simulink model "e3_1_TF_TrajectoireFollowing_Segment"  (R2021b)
settings: Solver=FixedStepAuto  StartTime=0.0  StopTime=100  FixedStep=sampleTime  RelTol=1e-3  EnableMultiTasking=on
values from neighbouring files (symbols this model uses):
  k_d_x = 1.5    [startSimulation.m]    (also in StartSimulation.m; start.m = 1.65)
  k_d_y = 1.5    [startSimulation.m]    (also in StartSimulation.m; start.m = 1.52)
  k_d_yaw = 1    [startSimulation.m]    (also in StartSimulation.m; start.m)
  k_d_z = 0.5    [startSimulation.m]    (also in StartSimulation.m; start.m)
  k_i_x = 0.01    [startSimulation.m]    (also in StartSimulation.m; start.m = 0.9)
  k_i_y = 0.01    [startSimulation.m]    (also in StartSimulation.m; start.m = 0.91)
  k_i_yaw = 0.01    [startSimulation.m]    (also in StartSimulation.m; start.m)
  k_i_z = 0.01    [startSimulation.m]    (also in StartSimulation.m; start.m)
  k_p_x = 1.2    [startSimulation.m]    (also in StartSimulation.m; start.m = 1.9)
  k_p_y = 1.5    [startSimulation.m]    (also in StartSimulation.m; start.m = 1.9)
  k_p_yaw = 2    [startSimulation.m]    (also in StartSimulation.m; start.m)
  k_p_z = 2    [startSimulation.m]    (also in StartSimulation.m; start.m)
  saturation_psi = 2    [startSimulation.m]    (also in StartSimulation.m; start.m)
  saturation_x = 2    [startSimulation.m]    (also in StartSimulation.m; start.m)
  saturation_y = 2    [startSimulation.m]    (also in StartSimulation.m; start.m)
  saturation_z = 2    [startSimulation.m]    (also in StartSimulation.m; start.m)
libraries: simulink x28, aerolibanimutils x1

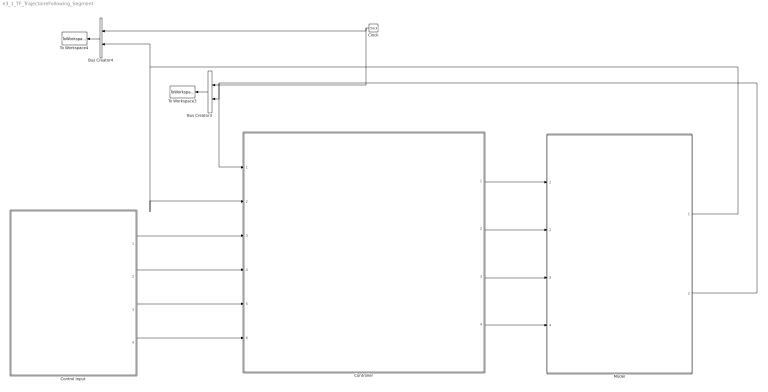
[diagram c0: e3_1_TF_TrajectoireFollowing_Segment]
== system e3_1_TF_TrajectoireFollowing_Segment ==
  Bus Creator3 : BusCreator  Inputs=2
  Bus Creator4 : BusCreator  Inputs=2
  Clock : Clock
  Control Input : Subsystem
  Controller : Subsystem
  Model : Subsystem
  To Workspace3 : ToWorkspace  VariableName=r1_pos_array  SampleTime=-1
  To Workspace4 : ToWorkspace  VariableName=r1_vel_array  SampleTime=-1
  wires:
  Clock/1 -> Bus Creator4/1, Bus Creator3/1
  Bus Creator3/1 -> To Workspace3/1
  Bus Creator4/1 -> To Workspace4/1
  Controller/1(Controller Output X) -> Model/1(Commande Input X)
  Controller/2(Controller Output Y) -> Model/2(Commande Input Y)
  Controller/3(Controller Output H) -> Model/3(Commande Input H)
  Controller/4(Controller Output Psi) -> Model/4(Commande Input Psi)
  Control Input/1(ux) -> Controller/3(Control input X)
  Control Input/2(uy) -> Controller/4(Control input Y)
  Control Input/3(uz) -> Controller/5(Control input H)
  Control Input/4(upsi) -> Controller/6(Control input Psi)
  Model/2(Output Position) -> Controller/1(Feedback Position), Bus Creator3/2
  Model/1(Output Velocity) -> Controller/2(Feedback Velocity), Bus Creator4/2

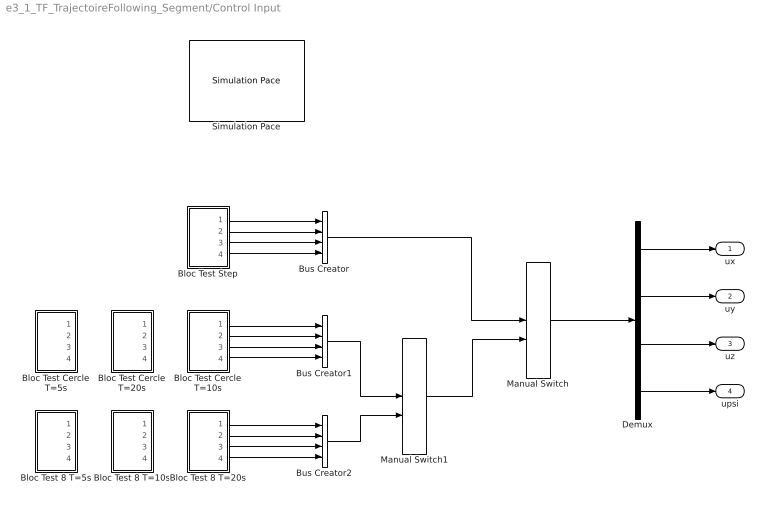
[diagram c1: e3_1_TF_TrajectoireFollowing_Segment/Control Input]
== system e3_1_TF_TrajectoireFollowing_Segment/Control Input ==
  Bloc Test 8 T=10s : Subsystem
  Bloc Test 8 T=20s : Subsystem
  Bloc Test 8 T=5s : Subsystem
  Bloc Test Cercle T=10s : Subsystem
  Bloc Test Cercle T=20s : Subsystem
  Bloc Test Cercle T=5s : Subsystem
  Bloc Test Step : Subsystem
  Bus Creator : BusCreator  Inputs=4
  Bus Creator1 : BusCreator  Inputs=4
  Bus Creator2 : BusCreator  Inputs=4
  Demux : Demux
  Manual Switch : ManualSwitch  CurrentSetting=0
  Manual Switch1 : ManualSwitch
  Simulation Pace : aerolibanimutils/Simulation Pace  SimulationPace=100  SleepMode=MATLAB Thread  OutputPaceError=off  SampleTime=-1
  ux : Outport  VectorParamsAs1DForOutWhenUnconnected=off
  uy : Outport  Port=2  VectorParamsAs1DForOutWhenUnconnected=off
  uz : Outport  Port=3  VectorParamsAs1DForOutWhenUnconnected=off
  upsi : Outport  Port=4  VectorParamsAs1DForOutWhenUnconnected=off
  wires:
  Demux/2 -> uy/1
  Demux/1 -> ux/1
  Bloc Test Step/2(uy) -> Bus Creator/2
  Demux/3 -> uz/1
  Demux/4 -> upsi/1
  Bloc Test Step/4(upsi) -> Bus Creator/4
  Bloc Test Step/3(uz) -> Bus Creator/3
  Bloc Test Step/1(ux) -> Bus Creator/1
  Bus Creator/1 -> Manual Switch/1
  Bloc Test Cercle T=10s/1(ux) -> Bus Creator1/1
  Bloc Test Cercle T=10s/4(upsi) -> Bus Creator1/4
  Bloc Test Cercle T=10s/2(uy) -> Bus Creator1/2
  Bloc Test Cercle T=10s/3(uz) -> Bus Creator1/3
  Bus Creator1/1 -> Manual Switch1/1
  Bloc Test 8 T=20s/1(ux) -> Bus Creator2/1
  Bloc Test 8 T=20s/2(uy) -> Bus Creator2/2
  Bloc Test 8 T=20s/3(uz) -> Bus Creator2/3
  Bloc Test 8 T=20s/4(upsi) -> Bus Creator2/4
  Bus Creator2/1 -> Manual Switch1/2
  Manual Switch/1 -> Demux/1
  Manual Switch1/1 -> Manual Switch/2

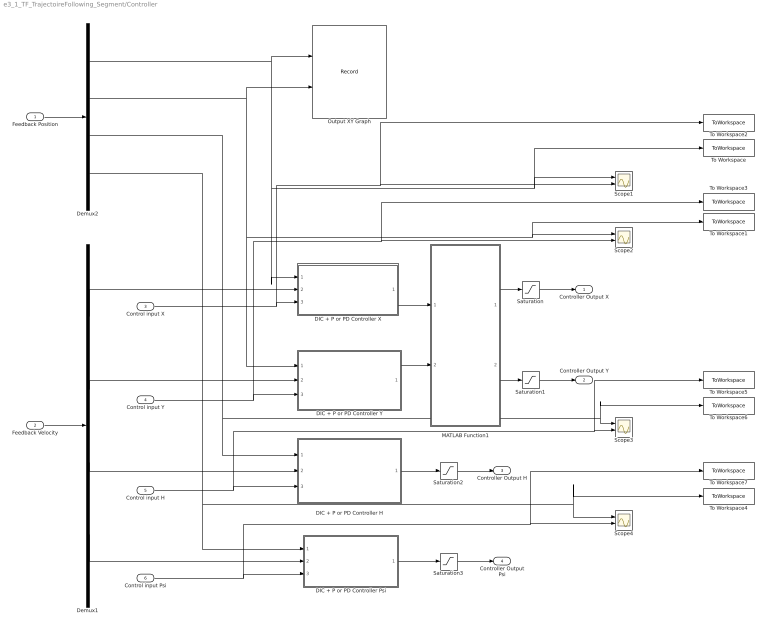
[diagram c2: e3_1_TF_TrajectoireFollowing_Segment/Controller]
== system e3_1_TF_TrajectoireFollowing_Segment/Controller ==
  Feedback Position : Inport
  Feedback Velocity : Inport  Port=2
  Control input X : Inport  Port=3
  Control input Y : Inport  Port=4
  Control input H : Inport  Port=5
  Control input Psi : Inport  Port=6
  DIC + P or PD Controller H : Subsystem
  DIC + P or PD Controller Psi : Subsystem
  DIC + P or PD Controller X : Subsystem
  DIC + P or PD Controller Y : Subsystem
  Demux1 : Demux
  Demux2 : Demux
  MATLAB Function1 : MATLAB Function  TreatAsAtomicUnit=on
  Output XY Graph : Record  Commented=on  FileSettingsInternal="{\"entries\":[{\"content\":{\"excelSettings\":{\"content\":{},\"type\":\"Streamout.ExcelSettings\"}},\"type\":\"Streamout.FileSettingStorage\",\"uuid\":\"257411f7-08c1-4fe0-ac72-024b6feac48e\"}],\"packageUris\":[\"http://schema.mathworks.com/mf0/streamout_blocks/R2020a\"],\"version\":\"1.0\"}"  Layout=[1 1]  SignalsInternal="{\"entries\":[{\"content\":{\"signals\":[{\"content\":{\"blockPath\":[\"e3_1_TF_TrajectoireFollowing_Segment/Controller/Output XY Graph\"],\"channel\":[],\"dimensions\":[1],\"domain\":\"e3_1_TF_TrajectoireFollowing_Segment/Controller/Output XY Graph\",\"lineColor\":\"#a2142f\",\"plots\":[1],\"port\":1,\"sid\":[],\"signalID\":73,\"signalName\":\"XY Graph:1\"},\"type\":\"RecordBlkView.Signal\",\"uuid\":\"3b188984-56d2-4a2b-b69d-3f50a3018f85\"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"  VisualizationBindings="{\"xyplotplugin\":{\"info\":[{\"series\":[{\"bindingParametersList\":[{\"parameter\":\"X-Axis\",\"signalID\":73,\"signalName\":\"XY Graph:1\"},{\"parameter\":\"Y-Axis\",\"signalID\":76,\"signalName\":\"XY Graph:2\"}],\"seriesID\":49033}],\"subplotID\":1}]}}"  CompatibilityTag=XY  st=-1
  Saturation : Saturate  UpperLimit=saturation_x  LowerLimit=-saturation_x
  Saturation1 : Saturate  UpperLimit=saturation_y  LowerLimit=-saturation_y
  Saturation2 : Saturate  UpperLimit=saturation_z  LowerLimit=-saturation_z
  Saturation3 : Saturate  UpperLimit=saturation_psi  LowerLimit=-saturation_psi
  Scope{1..4} (4 alike) : Scope  NumInputPorts=2
  To Workspace : ToWorkspace  VariableName=N4_Step1_Out_X  SampleTime=-1
  To Workspace1 : ToWorkspace  VariableName=N4_Step1_Out_Y  SampleTime=-1
  To Workspace2 : ToWorkspace  VariableName=N4_Step1_In_X  SampleTime=-1
  To Workspace3 : ToWorkspace  VariableName=N4_Step1_In_Y  SampleTime=-1
  To Workspace4 : ToWorkspace  VariableName=N4_Step1_Out_Psi  SampleTime=-1
  To Workspace5 : ToWorkspace  VariableName=N4_Step1_In_H  SampleTime=-1
  To Workspace6 : ToWorkspace  VariableName=N4_Step1_Out_H  SampleTime=-1
  To Workspace7 : ToWorkspace  VariableName=N4_Step1_In_Psi  SampleTime=-1
  Controller Output X : Outport  VectorParamsAs1DForOutWhenUnconnected=off
  Controller Output Y : Outport  Port=2  VectorParamsAs1DForOutWhenUnconnected=off
  Controller Output H : Outport  Port=3  VectorParamsAs1DForOutWhenUnconnected=off
  Controller Output Psi : Outport  Port=4  VectorParamsAs1DForOutWhenUnconnected=off
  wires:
  Feedback Position/1 -> Demux2/1
  Feedback Velocity/1 -> Demux1/1
  Demux1/2 -> DIC + P or PD Controller Y/2(Feedback Velocity Y)
  Demux2/3 -> Scope3/1, To Workspace6/1, DIC + P or PD Controller H/1(Feedback Position H)
  Demux1/1 -> DIC + P or PD Controller X/2(Feedback Velocity X)
  Demux1/3 -> DIC + P or PD Controller H/2(Feedback Velocity H)
  Control input X/1 -> To Workspace2/1, Scope1/2, DIC + P or PD Controller X/3(Control Input X)
  Control input H/1 -> Scope3/2, To Workspace5/1, DIC + P or PD Controller H/3(Control Input H)
  Saturation/1 -> Controller Output X/1
  Saturation1/1 -> Controller Output Y/1
  Saturation2/1 -> Controller Output H/1
  Saturation3/1 -> Controller Output Psi/1
  Control input Y/1 -> Scope2/2, To Workspace3/1, DIC + P or PD Controller Y/3(Control Input Y)
  DIC + P or PD Controller H/1(Controller Output H) -> Saturation2/1
  DIC + P or PD Controller Psi/1(Controller Output Psi) -> Saturation3/1
  Demux2/1 -> DIC + P or PD Controller X/1(Feedback Position X), To Workspace/1, Scope1/1, Output XY Graph/1
  Demux2/2 -> Scope2/1, To Workspace1/1, DIC + P or PD Controller Y/1(Feedback Position Y), Output XY Graph/2
  Demux2/4 -> Scope4/1, To Workspace4/1, DIC + P or PD Controller Psi/1(Feedback Position Psi)
  Demux1/4 -> DIC + P or PD Controller Psi/2(Feedback Velocity Psi)
  Control input Psi/1 -> Scope4/2, To Workspace7/1, DIC + P or PD Controller Psi/3(Control input Psi)
  DIC + P or PD Controller Y/1(Controller Output Y) -> MATLAB Function1/2(eay)
  MATLAB Function1/2(phi) -> Saturation1/1
  DIC + P or PD Controller X/1(Controller Output X) -> MATLAB Function1/1(eax)
  MATLAB Function1/1(theta) -> Saturation/1

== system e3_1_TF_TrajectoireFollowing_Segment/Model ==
  Commande Input X : Inport
  Commande Input Y : Inport  Port=2
  Commande Input H : Inport  Port=3
  Commande Input Psi : Inport  Port=4
  Step2_Model : Subsystem
  Output Velocity : Outport  VectorParamsAs1DForOutWhenUnconnected=off
  Output Position : Outport  Port=2  VectorParamsAs1DForOutWhenUnconnected=off
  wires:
  Commande Input Y/1 -> Step2_Model/2(In2)
  Commande Input Psi/1 -> Step2_Model/4(In4)
  Commande Input H/1 -> Step2_Model/3(In3)
  Step2_Model/1(Position) -> Output Position/1
  Commande Input X/1 -> Step2_Model/1(In1)
  Step2_Model/2(Velocity) -> Output Velocity/1

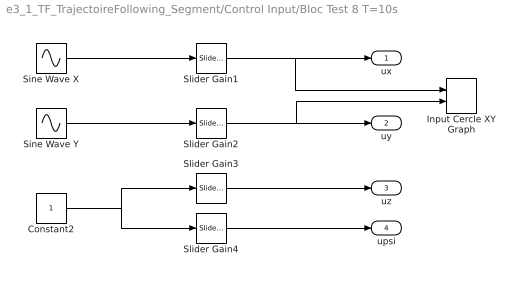
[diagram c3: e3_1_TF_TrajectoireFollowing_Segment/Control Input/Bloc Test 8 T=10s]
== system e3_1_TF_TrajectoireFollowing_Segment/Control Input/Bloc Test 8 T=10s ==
  Constant2 : Constant
  Input Cercle XY Graph : Record  Commented=on  FileSettingsInternal="{\"entries\":[{\"content\":{\"excelSettings\":{\"content\":{},\"type\":\"Streamout.ExcelSettings\"}},\"type\":\"Streamout.FileSettingStorage\",\"uuid\":\"03c5fa89-9371-4297-bf57-aca070f392fa\"}],\"packageUris\":[\"http://schema.mathworks.com/mf0/streamout_blocks/R2020a\"],\"version\":\"1.0\"}"  Layout=[1 1]  SignalsInternal="{\"entries\":[{\"content\":{\"signals\":[{\"content\":{\"blockPath\":[\"e3_1_TF_TrajectoireFollowing_Segment/Control Input/Bloc Test  8 T=10s/Input Cercle XY Graph\"],\"channel\":[],\"dimensions\":[1],\"domain\":\"e3_1_TF_TrajectoireFollowing_Segment/Control Input/Bloc Test  8 T=10s/Input Cercle XY Graph\",\"lineColor\":\"#a2142f\",\"plots\":[1],\"port\":1,\"sid\":[],\"signalID\":17,\"signalName\":\"XY Graph:1\"},\"type\":\"RecordBlkVi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"  VisualizationBindings="{\"xyplotplugin\":{\"info\":[{\"series\":[{\"bindingParametersList\":[{\"parameter\":\"X-Axis\",\"signalID\":17,\"signalName\":\"XY Graph:1\"},{\"parameter\":\"Y-Axis\",\"signalID\":20,\"signalName\":\"XY Graph:2\"}],\"seriesID\":13955}],\"subplotID\":1}]}}"  CompatibilityTag=XY  st=-1
  Sine Wave X : Sin  Frequency=0.65  SampleTime=0
  Sine Wave Y : Sin  Frequency=1.3  SampleTime=0
  Slider Gain1 : simulink/Math Operations/Slider Gain  gain=1  low=-10  high=10
  Slider Gain2 : simulink/Math Operations/Slider Gain  gain=1  low=-10  high=10
  Slider Gain3 : simulink/Math Operations/Slider Gain  gain=1  low=-3  high=3
  Slider Gain4 : simulink/Math Operations/Slider Gain  gain=0  low=-2  high=2
  ux : Outport  VectorParamsAs1DForOutWhenUnconnected=off
  uy : Outport  Port=2  VectorParamsAs1DForOutWhenUnconnected=off
  uz : Outport  Port=3  VectorParamsAs1DForOutWhenUnconnected=off
  upsi : Outport  Port=4  VectorParamsAs1DForOutWhenUnconnected=off
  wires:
  Slider Gain2/1 -> Input Cercle XY Graph/2, uy/1
  Slider Gain3/1 -> uz/1
  Slider Gain4/1 -> upsi/1
  Slider Gain1/1 -> Input Cercle XY Graph/1, ux/1
  Constant2/1 -> Slider Gain4/1, Slider Gain3/1
  Sine Wave Y/1 -> Slider Gain2/1
  Sine Wave X/1 -> Slider Gain1/1

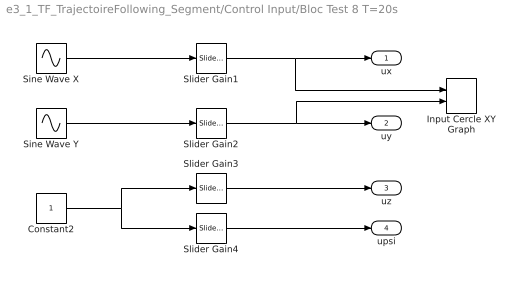
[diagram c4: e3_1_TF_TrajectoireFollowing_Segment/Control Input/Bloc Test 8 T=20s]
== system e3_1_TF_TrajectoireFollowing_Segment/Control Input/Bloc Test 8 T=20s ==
  Constant2 : Constant
  Input Cercle XY Graph : Record  Commented=on  FileSettingsInternal="{\"entries\":[{\"content\":{\"excelSettings\":{\"content\":{},\"type\":\"Streamout.ExcelSettings\"}},\"type\":\"Streamout.FileSettingStorage\",\"uuid\":\"e7845f50-59c4-48ea-8a84-4b8f90e03d5f\"}],\"packageUris\":[\"http://schema.mathworks.com/mf0/streamout_blocks/R2020a\"],\"version\":\"1.0\"}"  Layout=[1 1]  SignalsInternal="{\"entries\":[{\"content\":{\"signals\":[{\"content\":{\"blockPath\":[\"e3_1_TF_TrajectoireFollowing_Segment/Control Input/Bloc Test  8 T=20s/Input Cercle XY Graph\"],\"channel\":[],\"dimensions\":[1],\"domain\":\"e3_1_TF_TrajectoireFollowing_Segment/Control Input/Bloc Test  8 T=20s/Input Cercle XY Graph\",\"lineColor\":\"#a2142f\",\"plots\":[1],\"port\":1,\"sid\":[],\"signalID\":25,\"signalName\":\"XY Graph:1\"},\"type\":\"RecordBlkVi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"  VisualizationBindings="{\"xyplotplugin\":{\"info\":[{\"series\":[{\"bindingParametersList\":[{\"parameter\":\"X-Axis\",\"signalID\":25,\"signalName\":\"XY Graph:1\"},{\"parameter\":\"Y-Axis\",\"signalID\":28,\"signalName\":\"XY Graph:2\"}],\"seriesID\":39709}],\"subplotID\":1}]}}"  CompatibilityTag=XY  st=-1
  Sine Wave X : Sin  Frequency=0.35  SampleTime=0
  Sine Wave Y : Sin  Frequency=0.7  SampleTime=0
  Slider Gain1 : simulink/Math Operations/Slider Gain  gain=1  low=-10  high=10
  Slider Gain2 : simulink/Math Operations/Slider Gain  gain=1  low=-10  high=10
  Slider Gain3 : simulink/Math Operations/Slider Gain  gain=1  low=-3  high=3
  Slider Gain4 : simulink/Math Operations/Slider Gain  gain=0  low=-2  high=2
  ux : Outport  VectorParamsAs1DForOutWhenUnconnected=off
  uy : Outport  Port=2  VectorParamsAs1DForOutWhenUnconnected=off
  uz : Outport  Port=3  VectorParamsAs1DForOutWhenUnconnected=off
  upsi : Outport  Port=4  VectorParamsAs1DForOutWhenUnconnected=off
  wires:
  Slider Gain2/1 -> Input Cercle XY Graph/2, uy/1
  Slider Gain3/1 -> uz/1
  Slider Gain4/1 -> upsi/1
  Slider Gain1/1 -> Input Cercle XY Graph/1, ux/1
  Constant2/1 -> Slider Gain4/1, Slider Gain3/1
  Sine Wave Y/1 -> Slider Gain2/1
  Sine Wave X/1 -> Slider Gain1/1

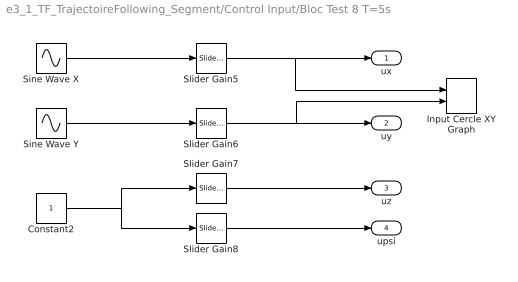
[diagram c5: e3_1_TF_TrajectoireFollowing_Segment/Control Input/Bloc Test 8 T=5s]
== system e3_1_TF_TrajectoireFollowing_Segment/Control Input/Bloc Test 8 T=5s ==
  Constant2 : Constant
  Input Cercle XY Graph : Record  Commented=on  FileSettingsInternal="{\"entries\":[{\"content\":{\"excelSettings\":{\"content\":{},\"type\":\"Streamout.ExcelSettings\"}},\"type\":\"Streamout.FileSettingStorage\",\"uuid\":\"b962c528-cdaa-49b8-a6b6-5a4193b1445c\"}],\"packageUris\":[\"http://schema.mathworks.com/mf0/streamout_blocks/R2020a\"],\"version\":\"1.0\"}"  Layout=[1 1]  SignalsInternal="{\"entries\":[{\"content\":{\"signals\":[{\"content\":{\"blockPath\":[\"e3_1_TF_TrajectoireFollowing_Segment/Control Input/Bloc Test  8 T=5s/Input Cercle XY Graph\"],\"channel\":[],\"dimensions\":[1],\"domain\":\"e3_1_TF_TrajectoireFollowing_Segment/Control Input/Bloc Test  8 T=5s/Input Cercle XY Graph\",\"lineColor\":\"#a2142f\",\"plots\":[1],\"port\":1,\"sid\":[],\"signalID\":33,\"signalName\":\"XY Graph:1\"},\"type\":\"RecordBlkView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"  VisualizationBindings="{\"xyplotplugin\":{\"info\":[{\"series\":[{\"bindingParametersList\":[{\"parameter\":\"X-Axis\",\"signalID\":33,\"signalName\":\"XY Graph:1\"},{\"parameter\":\"Y-Axis\",\"signalID\":36,\"signalName\":\"XY Graph:2\"}],\"seriesID\":55144}],\"subplotID\":1}]}}"  CompatibilityTag=XY  st=-1
  Sine Wave X : Sin  SampleTime=0
  Sine Wave Y : Sin  Frequency=2  SampleTime=0
  Slider Gain5 : simulink/Math Operations/Slider Gain  gain=1  low=-10  high=10
  Slider Gain6 : simulink/Math Operations/Slider Gain  gain=1  low=-10  high=10
  Slider Gain7 : simulink/Math Operations/Slider Gain  gain=1  low=-3  high=3
  Slider Gain8 : simulink/Math Operations/Slider Gain  gain=0  low=-2  high=2
  ux : Outport  VectorParamsAs1DForOutWhenUnconnected=off
  uy : Outport  Port=2  VectorParamsAs1DForOutWhenUnconnected=off
  uz : Outport  Port=3  VectorParamsAs1DForOutWhenUnconnected=off
  upsi : Outport  Port=4  VectorParamsAs1DForOutWhenUnconnected=off
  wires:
  Slider Gain6/1 -> Input Cercle XY Graph/2, uy/1
  Slider Gain7/1 -> uz/1
  Slider Gain8/1 -> upsi/1
  Slider Gain5/1 -> Input Cercle XY Graph/1, ux/1
  Constant2/1 -> Slider Gain8/1, Slider Gain7/1
  Sine Wave Y/1 -> Slider Gain6/1
  Sine Wave X/1 -> Slider Gain5/1

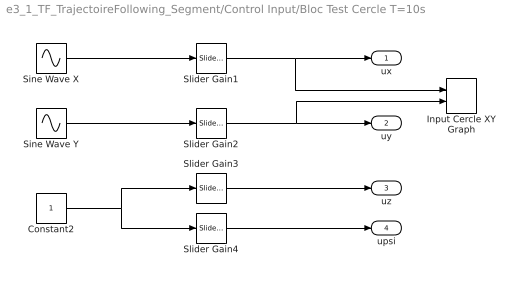
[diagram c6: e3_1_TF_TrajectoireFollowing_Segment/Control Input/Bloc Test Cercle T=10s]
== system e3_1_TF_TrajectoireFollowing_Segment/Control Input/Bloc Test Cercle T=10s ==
  Constant2 : Constant
  Input Cercle XY Graph : Record  Commented=on  FileSettingsInternal="{\"entries\":[{\"content\":{\"excelSettings\":{\"content\":{},\"type\":\"Streamout.ExcelSettings\"}},\"type\":\"Streamout.FileSettingStorage\",\"uuid\":\"4747c779-31ca-4c22-85fd-a8688f0d7ce9\"}],\"packageUris\":[\"http://schema.mathworks.com/mf0/streamout_blocks/R2020a\"],\"version\":\"1.0\"}"  Layout=[1 1]  SignalsInternal="{\"entries\":[{\"content\":{\"signals\":[{\"content\":{\"blockPath\":[\"e3_1_TF_TrajectoireFollowing_Segment/Control Input/Bloc Test  Cercle T=10s/Input Cercle XY Graph\"],\"channel\":[],\"dimensions\":[1],\"domain\":\"e3_1_TF_TrajectoireFollowing_Segment/Control Input/Bloc Test  Cercle T=10s/Input Cercle XY Graph\",\"lineColor\":\"#a2142f\",\"plots\":[1],\"port\":1,\"sid\":[],\"signalID\":41,\"signalName\":\"XY Graph:1\"},\"type\":\"R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"  VisualizationBindings="{\"xyplotplugin\":{\"info\":[{\"series\":[{\"bindingParametersList\":[{\"parameter\":\"X-Axis\",\"signalID\":41,\"signalName\":\"XY Graph:1\"},{\"parameter\":\"Y-Axis\",\"signalID\":44,\"signalName\":\"XY Graph:2\"}],\"seriesID\":10230}],\"subplotID\":1}]}}"  CompatibilityTag=XY  st=-1
  Sine Wave X : Sin  Frequency=0.65  SampleTime=0
  Sine Wave Y : Sin  Frequency=0.65  Phase=pi/2  SampleTime=0
  Slider Gain1 : simulink/Math Operations/Slider Gain  gain=1  low=-10  high=10
  Slider Gain2 : simulink/Math Operations/Slider Gain  gain=1  low=-10  high=10
  Slider Gain3 : simulink/Math Operations/Slider Gain  gain=1  low=-3  high=3
  Slider Gain4 : simulink/Math Operations/Slider Gain  gain=0  low=-2  high=2
  ux : Outport  VectorParamsAs1DForOutWhenUnconnected=off
  uy : Outport  Port=2  VectorParamsAs1DForOutWhenUnconnected=off
  uz : Outport  Port=3  VectorParamsAs1DForOutWhenUnconnected=off
  upsi : Outport  Port=4  VectorParamsAs1DForOutWhenUnconnected=off
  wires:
  Slider Gain2/1 -> Input Cercle XY Graph/2, uy/1
  Slider Gain3/1 -> uz/1
  Slider Gain4/1 -> upsi/1
  Slider Gain1/1 -> Input Cercle XY Graph/1, ux/1
  Constant2/1 -> Slider Gain4/1, Slider Gain3/1
  Sine Wave Y/1 -> Slider Gain2/1
  Sine Wave X/1 -> Slider Gain1/1

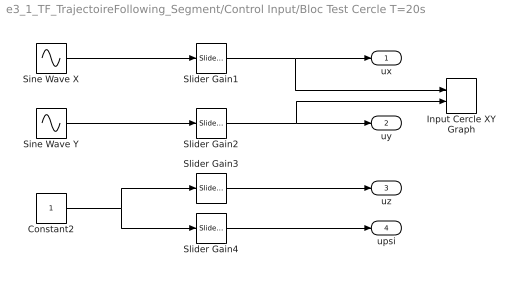
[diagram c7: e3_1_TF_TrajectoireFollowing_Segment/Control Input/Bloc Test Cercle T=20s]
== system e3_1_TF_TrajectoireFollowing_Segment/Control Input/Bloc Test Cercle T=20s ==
  Constant2 : Constant
  Input Cercle XY Graph : Record  Commented=on  FileSettingsInternal="{\"entries\":[{\"content\":{\"excelSettings\":{\"content\":{},\"type\":\"Streamout.ExcelSettings\"}},\"type\":\"Streamout.FileSettingStorage\",\"uuid\":\"72da48eb-6662-417d-afce-a372059077c8\"}],\"packageUris\":[\"http://schema.mathworks.com/mf0/streamout_blocks/R2020a\"],\"version\":\"1.0\"}"  Layout=[1 1]  SignalsInternal="{\"entries\":[{\"content\":{\"signals\":[{\"content\":{\"blockPath\":[\"e3_1_TF_TrajectoireFollowing_Segment/Control Input/Bloc Test  Cercle T=20s/Input Cercle XY Graph\"],\"channel\":[],\"dimensions\":[1],\"domain\":\"e3_1_TF_TrajectoireFollowing_Segment/Control Input/Bloc Test  Cercle T=20s/Input Cercle XY Graph\",\"lineColor\":\"#a2142f\",\"plots\":[1],\"port\":1,\"sid\":[],\"signalID\":49,\"signalName\":\"XY Graph:1\"},\"type\":\"R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"  VisualizationBindings="{\"xyplotplugin\":{\"info\":[{\"series\":[{\"bindingParametersList\":[{\"parameter\":\"X-Axis\",\"signalID\":49,\"signalName\":\"XY Graph:1\"},{\"parameter\":\"Y-Axis\",\"signalID\":52,\"signalName\":\"XY Graph:2\"}],\"seriesID\":7019}],\"subplotID\":1}]}}"  CompatibilityTag=XY  st=-1
  Sine Wave X : Sin  Frequency=0.35  SampleTime=0
  Sine Wave Y : Sin  Frequency=0.35  Phase=pi/2  SampleTime=0
  Slider Gain1 : simulink/Math Operations/Slider Gain  gain=1  low=-10  high=10
  Slider Gain2 : simulink/Math Operations/Slider Gain  gain=1  low=-10  high=10
  Slider Gain3 : simulink/Math Operations/Slider Gain  gain=1  low=-3  high=3
  Slider Gain4 : simulink/Math Operations/Slider Gain  gain=0  low=-2  high=2
  ux : Outport  VectorParamsAs1DForOutWhenUnconnected=off
  uy : Outport  Port=2  VectorParamsAs1DForOutWhenUnconnected=off
  uz : Outport  Port=3  VectorParamsAs1DForOutWhenUnconnected=off
  upsi : Outport  Port=4  VectorParamsAs1DForOutWhenUnconnected=off
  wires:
  Slider Gain2/1 -> Input Cercle XY Graph/2, uy/1
  Slider Gain3/1 -> uz/1
  Slider Gain4/1 -> upsi/1
  Slider Gain1/1 -> Input Cercle XY Graph/1, ux/1
  Constant2/1 -> Slider Gain4/1, Slider Gain3/1
  Sine Wave Y/1 -> Slider Gain2/1
  Sine Wave X/1 -> Slider Gain1/1

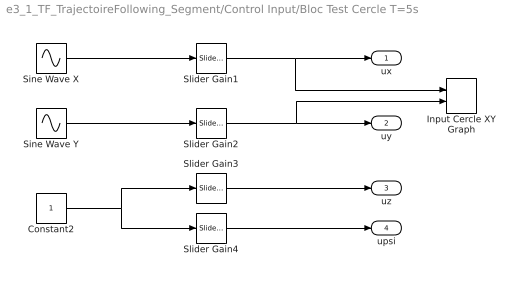
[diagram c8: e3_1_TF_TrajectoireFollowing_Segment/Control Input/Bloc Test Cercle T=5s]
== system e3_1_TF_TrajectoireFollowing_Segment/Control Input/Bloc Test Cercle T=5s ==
  Constant2 : Constant
  Input Cercle XY Graph : Record  Commented=on  FileSettingsInternal="{\"entries\":[{\"content\":{\"excelSettings\":{\"content\":{},\"type\":\"Streamout.ExcelSettings\"}},\"type\":\"Streamout.FileSettingStorage\",\"uuid\":\"f3cadc43-a327-48d7-aeff-f72ef859ed25\"}],\"packageUris\":[\"http://schema.mathworks.com/mf0/streamout_blocks/R2020a\"],\"version\":\"1.0\"}"  Layout=[1 1]  SignalsInternal="{\"entries\":[{\"content\":{\"signals\":[{\"content\":{\"blockPath\":[\"e3_1_TF_TrajectoireFollowing_Segment/Control Input/Bloc Test  Cercle T=5s/Input Cercle XY Graph\"],\"channel\":[],\"dimensions\":[1],\"domain\":\"e3_1_TF_TrajectoireFollowing_Segment/Control Input/Bloc Test  Cercle T=5s/Input Cercle XY Graph\",\"lineColor\":\"#a2142f\",\"plots\":[1],\"port\":1,\"sid\":[],\"signalID\":57,\"signalName\":\"XY Graph:1\"},\"type\":\"Rec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"  VisualizationBindings="{\"xyplotplugin\":{\"info\":[{\"series\":[{\"bindingParametersList\":[{\"parameter\":\"X-Axis\",\"signalID\":57,\"signalName\":\"XY Graph:1\"},{\"parameter\":\"Y-Axis\",\"signalID\":60,\"signalName\":\"XY Graph:2\"}],\"seriesID\":25171}],\"subplotID\":1}]}}"  CompatibilityTag=XY  st=-1
  Sine Wave X : Sin  SampleTime=0
  Sine Wave Y : Sin  Phase=pi/2  SampleTime=0
  Slider Gain1 : simulink/Math Operations/Slider Gain  gain=1  low=-10  high=10
  Slider Gain2 : simulink/Math Operations/Slider Gain  gain=1  low=-10  high=10
  Slider Gain3 : simulink/Math Operations/Slider Gain  gain=1  low=-3  high=3
  Slider Gain4 : simulink/Math Operations/Slider Gain  gain=0  low=-2  high=2
  ux : Outport  VectorParamsAs1DForOutWhenUnconnected=off
  uy : Outport  Port=2  VectorParamsAs1DForOutWhenUnconnected=off
  uz : Outport  Port=3  VectorParamsAs1DForOutWhenUnconnected=off
  upsi : Outport  Port=4  VectorParamsAs1DForOutWhenUnconnected=off
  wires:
  Slider Gain2/1 -> Input Cercle XY Graph/2, uy/1
  Slider Gain3/1 -> uz/1
  Slider Gain4/1 -> upsi/1
  Slider Gain1/1 -> Input Cercle XY Graph/1, ux/1
  Constant2/1 -> Slider Gain4/1, Slider Gain3/1
  Sine Wave Y/1 -> Slider Gain2/1
  Sine Wave X/1 -> Slider Gain1/1

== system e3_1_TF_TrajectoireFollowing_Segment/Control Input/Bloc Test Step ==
  Constant2 : Constant
  Input Segment XY Graph : Record  Commented=on  FileSettingsInternal="{\"entries\":[{\"content\":{\"excelSettings\":{\"content\":{},\"type\":\"Streamout.ExcelSettings\"}},\"type\":\"Streamout.FileSettingStorage\",\"uuid\":\"6e8eea62-37b8-4598-ade1-409acda76b02\"}],\"packageUris\":[\"http://schema.mathworks.com/mf0/streamout_blocks/R2020a\"],\"version\":\"1.0\"}"  Layout=[1 1]  SignalsInternal="{\"entries\":[{\"content\":{\"signals\":[{\"content\":{\"blockPath\":[\"e3_1_TF_TrajectoireFollowing_Segment/Control Input/Bloc Test  Step/Input Segment XY Graph\"],\"channel\":[],\"dimensions\":[1],\"domain\":\"e3_1_TF_TrajectoireFollowing_Segment/Control Input/Bloc Test  Step/Input Segment XY Graph\",\"lineColor\":\"#a2142f\",\"plots\":[1],\"port\":1,\"sid\":[],\"signalID\":65,\"signalName\":\"XY Graph:1\"},\"type\":\"RecordBlkView.S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"  VisualizationBindings="{\"xyplotplugin\":{\"info\":[{\"series\":[{\"bindingParametersList\":[{\"parameter\":\"X-Axis\",\"signalID\":65,\"signalName\":\"XY Graph:1\"},{\"parameter\":\"Y-Axis\",\"signalID\":68,\"signalName\":\"XY Graph:2\"}],\"seriesID\":8843}],\"subplotID\":1}]}}"  CompatibilityTag=XY  st=-1
  Slider Gain1 : simulink/Math Operations/Slider Gain  gain=1  low=-10  high=10
  Slider Gain2 : simulink/Math Operations/Slider Gain  gain=1  low=-10  high=10
  Slider Gain3 : simulink/Math Operations/Slider Gain  gain=1  low=-2  high=2
  Slider Gain4 : simulink/Math Operations/Slider Gain  gain=0  low=-2  high=2
  Step X1 : Step  Time=5  SampleTime=0
  ux : Outport  VectorParamsAs1DForOutWhenUnconnected=off
  uy : Outport  Port=2  VectorParamsAs1DForOutWhenUnconnected=off
  uz : Outport  Port=3  VectorParamsAs1DForOutWhenUnconnected=off
  upsi : Outport  Port=4  VectorParamsAs1DForOutWhenUnconnected=off
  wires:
  Slider Gain1/1 -> Input Segment XY Graph/1, ux/1
  Slider Gain2/1 -> Input Segment XY Graph/2, uy/1
  Slider Gain3/1 -> uz/1
  Slider Gain4/1 -> upsi/1
  Step X1/1 -> Slider Gain3/1, Slider Gain4/1, Slider Gain2/1, Slider Gain1/1

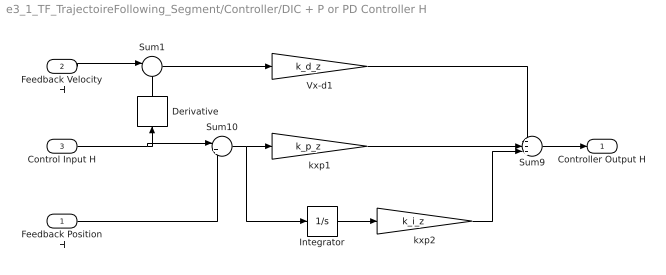
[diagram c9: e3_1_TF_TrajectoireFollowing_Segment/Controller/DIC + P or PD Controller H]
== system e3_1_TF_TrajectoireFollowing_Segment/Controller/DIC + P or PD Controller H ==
  Feedback Position H : Inport
  Feedback Velocity H : Inport  Port=2
  Control Input H : Inport  Port=3
  Derivative : Derivative
  Integrator : Integrator
  Sum1 : Sum  Inputs=|-+
  Sum10 : Sum  Inputs=|+-
  Sum9 : Sum  Inputs=+++|
  Vx-d1 : Gain  Gain=k_d_z
  kxp1 : Gain  Gain=k_p_z
  kxp2 : Gain  Gain=k_i_z
  Controller Output H : Outport  VectorParamsAs1DForOutWhenUnconnected=off
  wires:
  Sum9/1 -> Controller Output H/1
  Sum10/1 -> Integrator/1, kxp1/1
  kxp1/1 -> Sum9/2
  Vx-d1/1 -> Sum9/1
  Feedback Velocity H/1 -> Sum1/1
  Sum1/1 -> Vx-d1/1
  Integrator/1 -> kxp2/1
  kxp2/1 -> Sum9/3
  Control Input H/1 -> Sum10/1, Derivative/1
  Feedback Position H/1 -> Sum10/2
  Derivative/1 -> Sum1/2

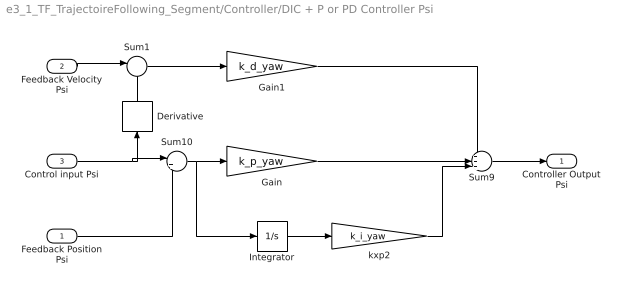
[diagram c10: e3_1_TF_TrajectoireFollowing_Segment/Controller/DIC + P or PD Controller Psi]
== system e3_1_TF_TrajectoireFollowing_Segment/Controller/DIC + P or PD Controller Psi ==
  Feedback Position Psi : Inport
  Feedback Velocity Psi : Inport  Port=2
  Control input Psi : Inport  Port=3
  Derivative : Derivative
  Gain : Gain  Gain=k_p_yaw
  Gain1 : Gain  Gain=k_d_yaw
  Integrator : Integrator
  Sum1 : Sum  Inputs=|-+
  Sum10 : Sum  Inputs=|+-
  Sum9 : Sum  Inputs=+++|
  kxp2 : Gain  Gain=k_i_yaw
  Controller Output Psi : Outport  VectorParamsAs1DForOutWhenUnconnected=off
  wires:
  Sum9/1 -> Controller Output Psi/1
  kxp2/1 -> Sum9/3
  Control input Psi/1 -> Sum10/1, Derivative/1
  Gain1/1 -> Sum9/1
  Sum10/1 -> Gain/1, Integrator/1
  Integrator/1 -> kxp2/1
  Feedback Velocity Psi/1 -> Sum1/1
  Sum1/1 -> Gain1/1
  Gain/1 -> Sum9/2
  Derivative/1 -> Sum1/2
  Feedback Position Psi/1 -> Sum10/2

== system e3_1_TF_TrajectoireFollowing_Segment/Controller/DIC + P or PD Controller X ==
  Feedback Position X : Inport
  Feedback Velocity X : Inport  Port=2
  Control Input X : Inport  Port=3
  Derivative : Derivative
  Integrator : Integrator
  Sum1 : Sum  Inputs=|-+
  Sum10 : Sum  Inputs=|+-
  Sum9 : Sum  Inputs=+++|
  Vx-d3 : Gain  Gain=k_d_x
  kxp2 : Gain  Gain=k_i_x
  kxp3 : Gain  Gain=k_p_x
  Controller Output X : Outport  VectorParamsAs1DForOutWhenUnconnected=off
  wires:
  Sum9/1 -> Controller Output X/1
  Feedback Velocity X/1 -> Sum1/1
  Feedback Position X/1 -> Sum10/2
  Sum1/1 -> Vx-d3/1
  Integrator/1 -> kxp2/1
  kxp3/1 -> Sum9/2
  Vx-d3/1 -> Sum9/1
  Sum10/1 -> kxp3/1, Integrator/1
  Derivative/1 -> Sum1/2
  kxp2/1 -> Sum9/3
  Control Input X/1 -> Sum10/1, Derivative/1

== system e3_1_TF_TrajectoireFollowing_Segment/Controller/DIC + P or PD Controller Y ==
  Feedback Position Y : Inport
  Feedback Velocity Y : Inport  Port=2
  Control Input Y : Inport  Port=3
  Derivative : Derivative
  Integrator : Integrator
  Sum1 : Sum  Inputs=|-+
  Sum10 : Sum  Inputs=|+-
  Sum9 : Sum  Inputs=+++|
  Vx-d3 : Gain  Gain=k_d_y
  kxp2 : Gain  Gain=k_i_y
  kxp3 : Gain  Gain=k_p_y
  Controller Output Y : Outport  VectorParamsAs1DForOutWhenUnconnected=off
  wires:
  Feedback Position Y/1 -> Sum10/2
  Control Input Y/1 -> Sum10/1, Derivative/1
  Sum9/1 -> Controller Output Y/1
  Integrator/1 -> kxp2/1
  kxp3/1 -> Sum9/2
  Sum10/1 -> kxp3/1, Integrator/1
  kxp2/1 -> Sum9/3
  Vx-d3/1 -> Sum9/1
  Feedback Velocity Y/1 -> Sum1/1
  Sum1/1 -> Vx-d3/1
  Derivative/1 -> Sum1/2

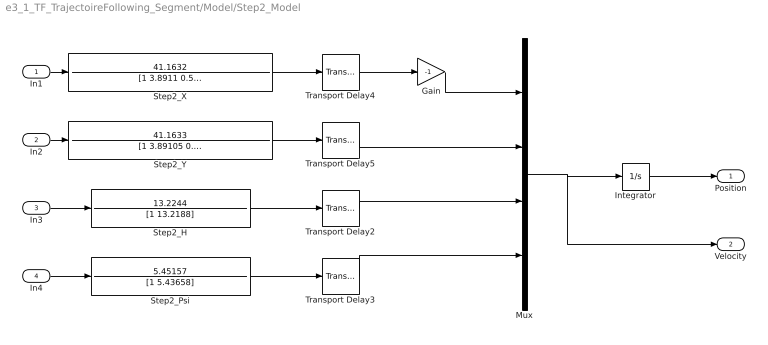
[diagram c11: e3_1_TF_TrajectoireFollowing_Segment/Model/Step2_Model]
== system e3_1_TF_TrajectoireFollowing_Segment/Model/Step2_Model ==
  In1 : Inport
  In2 : Inport  Port=2
  In3 : Inport  Port=3
  In4 : Inport  Port=4
  Gain : Gain  Gain=-1
  Integrator : Integrator
  Mux : Mux
  Step2_H : TransferFcn  Numerator=13.2244  Denominator=[1 13.2188]
  Step2_Psi : TransferFcn  Numerator=5.45157  Denominator=[1 5.43658]
  Step2_X : TransferFcn  Numerator=41.1632  Denominator=[1 3.8911 0.529635]
  Step2_Y : TransferFcn  Numerator=41.1633  Denominator=[1 3.89105 0.529839]
  Transport Delay2 : TransportDelay  DelayTime=0.0344
  Transport Delay3 : TransportDelay  DelayTime=0.0313
  Transport Delay4 : TransportDelay  DelayTime=0.0289
  Transport Delay5 : TransportDelay  DelayTime=0.0289
  Position : Outport  VectorParamsAs1DForOutWhenUnconnected=off
  Velocity : Outport  Port=2  VectorParamsAs1DForOutWhenUnconnected=off
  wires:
  Transport Delay2/1 -> Mux/3
  In2/1 -> Step2_Y/1
  In4/1 -> Step2_Psi/1
  Transport Delay3/1 -> Mux/4
  In1/1 -> Step2_X/1
  In3/1 -> Step2_H/1
  Step2_H/1 -> Transport Delay2/1
  Step2_Y/1 -> Transport Delay5/1
  Step2_X/1 -> Transport Delay4/1
  Step2_Psi/1 -> Transport Delay3/1
  Transport Delay4/1 -> Gain/1
  Transport Delay5/1 -> Mux/2
  Integrator/1 -> Position/1
  Mux/1 -> Velocity/1, Integrator/1
  Gain/1 -> Mux/1

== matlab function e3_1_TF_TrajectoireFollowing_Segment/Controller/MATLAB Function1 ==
function [theta,phi] = fcn(eax,eay)
g=9.8;

theta =-eax/g;% vx
phi =eay/g;% vy
